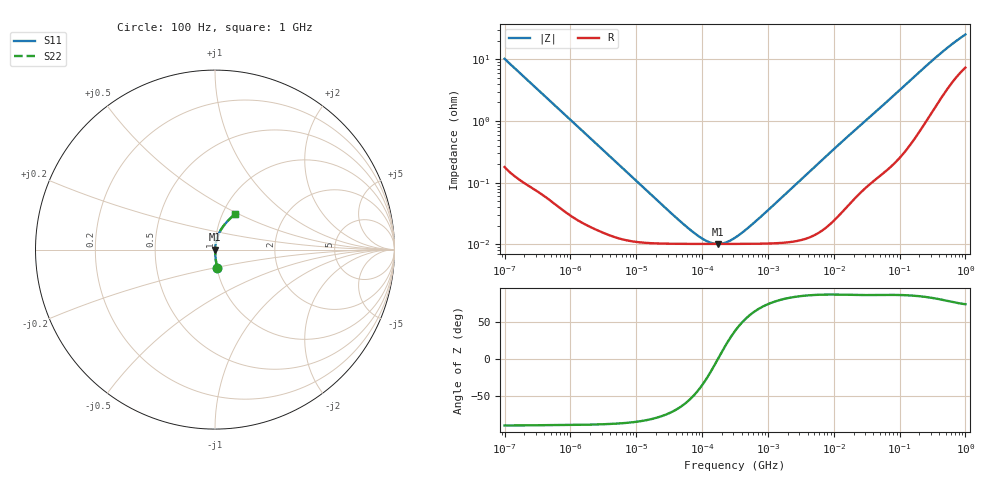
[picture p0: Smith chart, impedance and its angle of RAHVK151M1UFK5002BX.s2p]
! RAHVK151M1UFK5002BX  S-PARAMETER MODEL  (AEC-Q200 qualified)
! Model Generated by ELNA Corporation (http://www.ty-top.com)
! Version 1.0
! ELNA Control No. 240315
! Copyright (c) 20204 ELNA CO.,LTD. All Rights Reserved.
! Products Name : CONDUCTIVE POLYMER HYBRID ALUMINUM ELECTROLYTIC CAPACITORS
! Characteristics :
!  Capacitance  :  150uF  ,  Rated voltage  :  50V
!  Operating Temp. Range  :  -55 to +125 degC  ,  Endurance  :  6000hr at 125 degC
!  Dimension D  :  10mm  ,  Dimension L  :  12.5mm
! Frequency Range : 100Hz - 1GHz
! External Node Assignments :
!  1  o---| |---o  2
# MHz S RI R 50
!Freq[MHz].  S11 Real  S11 Imag  S21 Real  S21 Imag  S12 Real  S12 Imag  S22 Real  S22 Imag
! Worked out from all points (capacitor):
!   401 points, 100 Hz to 1 GHz, reference 50 ohm
!   read as one part in series: C = 156 uF near 108 Hz
!   lowest |Z| = 10.2 mohm at 172.8 kHz (marker M1)
!   series resonance near 174.3 kHz, so ESL is about 5.3 nH
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0.0001  0.012 -0.1005  0.988 0.1005  0.988 0.1005  0.012 -0.1005
0.000113  0.00963 -0.0893  0.9904 0.0893  0.9904 0.0893  0.00963 -0.0893
0.000183  0.00415 -0.0556  0.9959 0.0556  0.9959 0.0556  0.00415 -0.0556
0.000309  0.00183 -0.0332  0.9982 0.0332  0.9982 0.0332  0.00183 -0.0332
0.001488  0.000275 -0.00705  0.9997 0.00705  0.9997 0.00705  0.000275 -0.00705
0.022131  0.000104 -0.000476  0.9999 0.000476  0.9999 0.000476  0.000104 -0.000476
0.051582  0.000102 -0.000189  0.9999 0.000189  0.9999 0.000189  0.000102 -0.000189
0.087096  0.000102 -9.23e-05  0.9999 9.23e-05  0.9999 9.23e-05  0.000102 -9.23e-05
0.12517  0.000102 -4.14e-05  0.9999 4.14e-05  0.9999 4.14e-05  0.000102 -4.14e-05
0.147062  0.000102 -2.1e-05  0.9999 2.1e-05  0.9999 2.1e-05  0.000102 -2.1e-05
0.172783  0.000102 -1.05e-06  0.9999 1.05e-06  0.9999 1.05e-06  0.000102 -1.05e-06
0.229087  0.000102 3.41e-05  0.9999 -3.41e-05  0.9999 -3.41e-05  0.000102 3.41e-05
0.316228  0.000102 7.77e-05  0.9999 -7.77e-05  0.9999 -7.77e-05  0.000102 7.77e-05
0.436516  0.000102 0.000129  0.9999 -0.000129  0.9999 -0.000129  0.000102 0.000129
0.707946  0.000103 0.000235  0.9999 -0.000235  0.9999 -0.000235  0.000103 0.000235
4.704354  0.000138 0.00165  0.9999 -0.00165  0.9999 -0.00165  0.000138 0.00165
13.96368  0.000372 0.00481  0.9996 -0.00481  0.9996 -0.00481  0.000372 0.00481
69.9842  0.00222 0.0222  0.9978 -0.0222  0.9978 -0.0222  0.00222 0.0222
169.8244  0.00789 0.0521  0.9921 -0.0521  0.9921 -0.0521  0.00789 0.0521
380.1894  0.0308 0.107  0.9692 -0.107  0.9692 -0.107  0.0308 0.107
641.9482  0.0676 0.156  0.9324 -0.156  0.9324 -0.156  0.0676 0.156
1000  0.1134 0.1998  0.8866 -0.1998  0.8866 -0.1998  0.1134 0.1998
